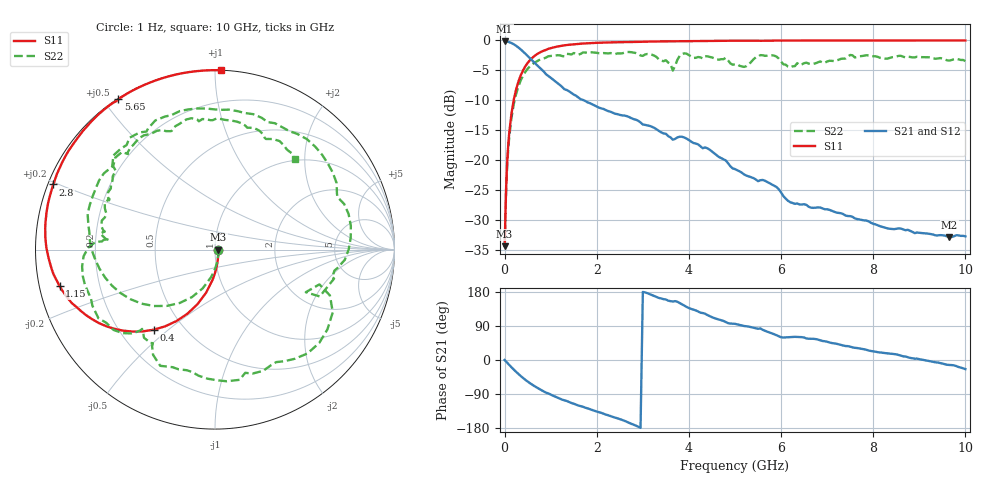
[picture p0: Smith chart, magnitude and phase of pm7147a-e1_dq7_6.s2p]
# GHz S DB R 50
! S-Parameters data
! Freq  dbS11  angS11  dbS21  angS21  dbS12  angS12  dbS22  angS22
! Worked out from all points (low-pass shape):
!   279 points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, 1 Hz to 10 GHz, reference 50 ohm
!   highest |S21| = -0.17 dB at 25.12 kHz (marker M1); lowest = -32.9 dB at 9.65 GHz (marker M2)
!   |S21| within 3 dB of the highest: start of sweep to 575.1 MHz
!   lowest |S11| = -34.4 dB at 19.95 kHz (marker M3), VSWR 1.04, Z = 51.9 - j0.00346 ohm
!   |S11| at or under -10 dB: start of sweep to 197.4 MHz
!   |S22| runs from -34.4 to -1.9 dB; largest |S21 - S12| = 0
!   S11 on the Smith chart (normalised r, x): 1 Hz: 1.04, -0.00; 400 MHz: 0.34, -0.45; 1.15 GHz: 0.06, -0.11; 2.8 GHz: 0.01, +0.19; 5.65 GHz: 0.00, +0.55; 10 GHz: 0.00, +1.03
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1e-09  -34.44 -0.0  -0.17 -0.0  -0.17 -0.0  -34.44 -0.0
1.99526e-05  -34.44 -0.1  -0.17 -0.0  -0.17 -0.0  -34.44 -0.1
2.51189e-05  -34.44 -0.1  -0.17 -0.0  -0.17 -0.0  -34.44 -0.1
0.03981072  -23.15 -78.2  -0.19 -5.2  -0.19 -5.2  -23.81 -78.6
0.1  -15.53 -94.4  -0.29 -13.0  -0.29 -13.0  -16.22 -98.0
0.4  -5.01 -127.4  -1.85 -47.5  -1.85 -47.5  -5.89 -143.6
0.75  -2.08 -150.5  -4.48 -76.2  -4.48 -76.2  -3.28 -179.5
1.15  -1.02 -166.8  -7.16 -99.3  -7.16 -99.3  -2.48 149.2
1.7  -0.52 178.2  -9.96 -123.4  -9.96 -123.4  -2.02 114.8
2.3  -0.33 166.2  -11.94 -148.1  -11.94 -148.1  -2.11 74.3
2.8  -0.25 158.1  -13.17 -170.8  -13.17 -170.8  -2.04 37.2
3.35  -0.17 150.1  -15.15 163.7  -15.15 163.7  -3.21 -8.5
3.65  -0.14 145.9  -16.61 154.3  -16.61 154.3  -5.06 -25.1
3.8  -0.14 144.0  -16.12 150.3  -16.12 150.3  -2.58 -28.0
4.35  -0.09 137.2  -17.91 122.2  -17.91 122.2  -2.64 -79.4
5.05  -0.04 129.0  -21.73 93.9  -21.73 93.9  -4.00 -128.9
5.65  -0.04 122.8  -23.49 77.1  -23.49 77.1  -2.58 -158.4
6  -0.02 119.2  -25.44 60.0  -25.44 60.0  -3.54 176.2
6.7  -0.01 112.6  -28.03 55.9  -28.03 55.9  -3.92 161.7
8.35  -0.00 99.1  -31.52 17.1  -31.52 17.1  -2.95 109.3
9.65  -0.00 90.3  -32.92 -13.1  -32.92 -13.1  -3.37 65.2
10  -0.00 88.1  -32.79 -24.2  -32.79 -24.2  -3.45 48.5
